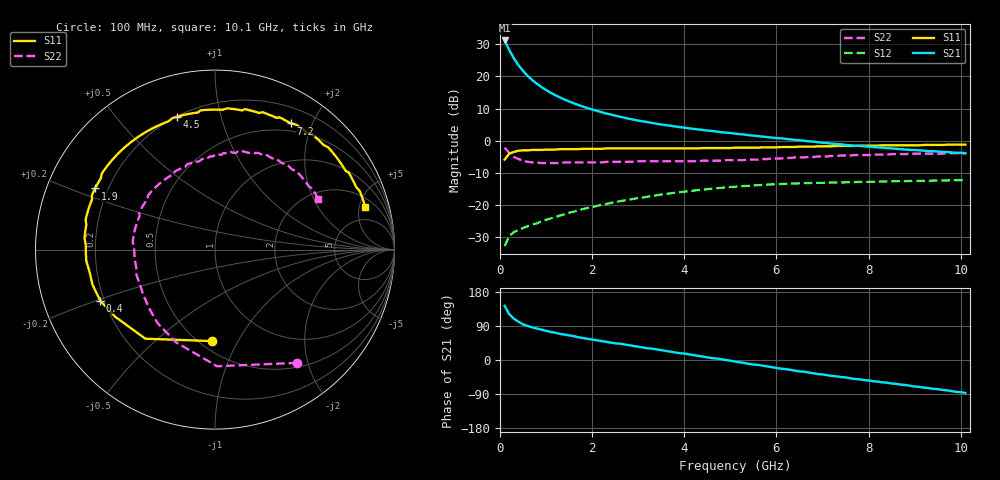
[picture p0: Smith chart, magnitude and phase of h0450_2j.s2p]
!HBFP-0450
!S and NOISE PARAMETERS at Vce=2V  Ic=100mA.  LAST UPDATED  09-04-98
# GHZ S MA R  50
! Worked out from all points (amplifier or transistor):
!   101 points, 100 MHz to 10.1 GHz, reference 50 ohm
!   highest |S21| = 31.2 dB at 100 MHz (marker M1)
!   |S21| within 3 dB of that: start of sweep to 201.1 MHz
!   unconditionally stable (mu >= 1): 1.898 GHz to end of sweep
!   at 1.7 GHz: K = 0.98, MSG = 16.4 dB, |S12| = -21.6 dB
!   at 5.1 GHz: K = 1.07, MAG = 6.6 dB, |S12| = -14.3 dB
!   at 10.1 GHz: K = 1.06, MAG = 2.7 dB, |S12| = -12.3 dB
!   lowest NFmin = 2.42 dB at 1.8 GHz
!   S11 on the Smith chart (normalised r, x): 100 MHz: 0.57, -0.79; 400 MHz: 0.18, -0.21; 1.9 GHz: 0.15, +0.23; 4.5 GHz: 0.20, +0.73; 7.2 GHz: 0.40, +1.70; 10.1 GHz: 2.88, +5.69
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0.1  0.51 -92.0  36.21 143.0  0.023 58.0  0.78 -54.0
0.2  0.63 -128.0  25.72 121.0  0.033 44.0  0.65 -89.0
0.3  0.67 -146.0  19.13 109.0  0.038 39.0  0.56 -113.0
0.4  0.7 -156.0  14.96 101.0  0.041 37.0  0.52 -128.0
0.5  0.71 -164.0  12.18 94.0  0.044 37.0  0.49 -139.0
0.6  0.71 -170.0  10.18 90.0  0.047 38.0  0.47 -149.0
0.7  0.72 -175.0  8.76 86.0  0.05 38.0  0.46 -156.0
0.8  0.72 -179.0  7.68 83.0  0.052 39.0  0.46 -162.0
0.9  0.72 178.0  6.83 80.0  0.056 40.0  0.45 -167.0
1.1  0.73 172.0  5.58 74.0  0.062 40.0  0.45 -175.0
1.3  0.74 167.0  4.72 69.0  0.069 41.0  0.45 178.0
1.5  0.74 162.0  4.08 65.0  0.076 40.0  0.46 172.0
1.8  0.75 156.0  3.4 58.0  0.087 39.0  0.46 164.0
1.9  0.75 153.0  3.22 56.0  0.09 38.0  0.46 162.0
2.5  0.76 142.0  2.46 44.0  0.111 34.0  0.47 150.0
3.5  0.76 124.0  1.79 26.0  0.146 23.0  0.48 133.0
4.5  0.77 106.0  1.44 7.0  0.177 10.0  0.49 115.0
5.1  0.78 96.0  1.29 -4.0  0.193 1.0  0.5 104.0
6.8  0.81 65.0  0.97 -35.0  0.221 -25.0  0.56 75.0
7.2  0.82 59.0  0.9 -42.0  0.224 -30.0  0.58 69.0
8.5  0.85 40.0  0.76 -62.0  0.234 -48.0  0.62 50.0
10.1  0.87 16.0  0.64 -87.0  0.244 -71.0  0.64 26.0
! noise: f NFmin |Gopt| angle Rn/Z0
1.8  2.42  0.68  -149  0.16
2  2.48  0.69  -147  0.18
2.5  2.61  0.69  -137  0.29
3.5  2.87  0.71  -120  0.6
4  3  0.74  -110  0.87
5  3.27  0.76  -92  1.46
5.5  3.4  0.78  -84  1.96
7  3.8  0.81  -57  3.73
8  4.06  0.83  -42  5.27
10  4.59  0.84  -14  8
